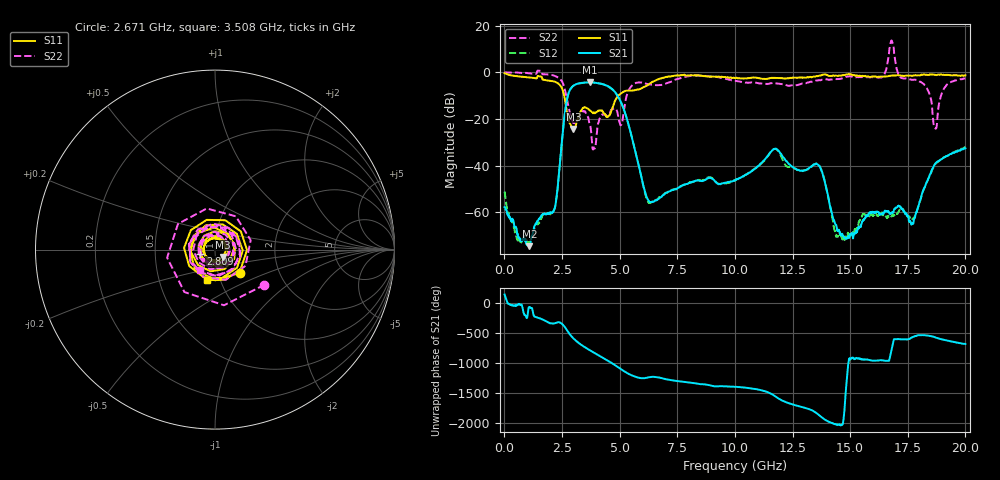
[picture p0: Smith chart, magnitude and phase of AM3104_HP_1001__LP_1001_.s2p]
!Created with skrf (http://scikit-rf.org).
# Hz S RI R 50.0
!freq ReS11 ImS11 ReS21 ImS21 ReS12 ImS12 ReS22 ImS22
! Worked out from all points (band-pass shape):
!   1601 points, 10 MHz to 20 GHz, reference 50 ohm
!   highest |S21| = -4.26 dB at 3.708 GHz (marker M1); lowest = -74.6 dB at 1.084 GHz (marker M2)
!   |S21| within 3 dB of the highest: 2.86 GHz to 4.683 GHz (1.823 GHz wide, 48.3 % of centre)
!   lowest |S11| = -24.3 dB at 2.996 GHz (marker M3), VSWR 1.13, Z = 54.5 - j4.55 ohm
!   |S11| at or under -10 dB: 2.594 GHz to 4.945 GHz (2.352 GHz wide, 62.4 % of centre)
!   |S22| runs from -33.1 to 13.7 dB; largest |S21 - S12| = 0.048
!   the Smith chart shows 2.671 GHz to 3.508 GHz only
!   S11 on the Smith chart (normalised r, x): 2.671 GHz: 1.27, -0.34; 2.809 GHz: 0.85, -0.04; 3.508 GHz: 0.86, -0.30
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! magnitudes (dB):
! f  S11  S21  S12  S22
! 10 MHz  -0.4  -57.9  -51.2  0.0
! 1.084 GHz  -2.2  -74.6  -73.1  -0.4
! 2.184 GHz  -4.0  -58.2  -58.4  -1.5
! 2.671 GHz  -14.5  -14.2  -14.2  -9.4
! 2.809 GHz  -21.3  -8.3  -8.3  -16.2
! 2.996 GHz  -24.3  -5.7  -5.7  -21.7
! 3.346 GHz  -16.2  -4.6  -4.6  -17.0
! 3.508 GHz  -15.1  -4.4  -4.5  -16.9
! 3.708 GHz  -16.3  -4.3  -4.3  -22.5
! 4.933 GHz  -10.1  -10.5  -10.5  -18.9
! 6.182 GHz  -5.7  -53.7  -54.4  -5.0
! 6.682 GHz  -3.0  -54.3  -54.1  -5.5
! 10.01 GHz  -2.5  -46.5  -46.3  -3.7
! 11.72 GHz  -2.4  -32.9  -33.0  -4.7
! 13.34 GHz  -2.1  -40.2  -40.3  -4.0
! 13.78 GHz  -1.1  -42.7  -42.5  -3.2
! 14.42 GHz  -1.5  -66.4  -70.2  -2.9
! 16.68 GHz  -1.6  -60.0  -62.0  7.3
! 17.71 GHz  -1.4  -64.9  -63.1  -3.2
! 18.69 GHz  -1.1  -39.3  -39.4  -24.0
! 19.11 GHz  -1.2  -36.4  -36.3  -6.4
! 20 GHz  -1.3  -32.6  -32.2  -2.6
